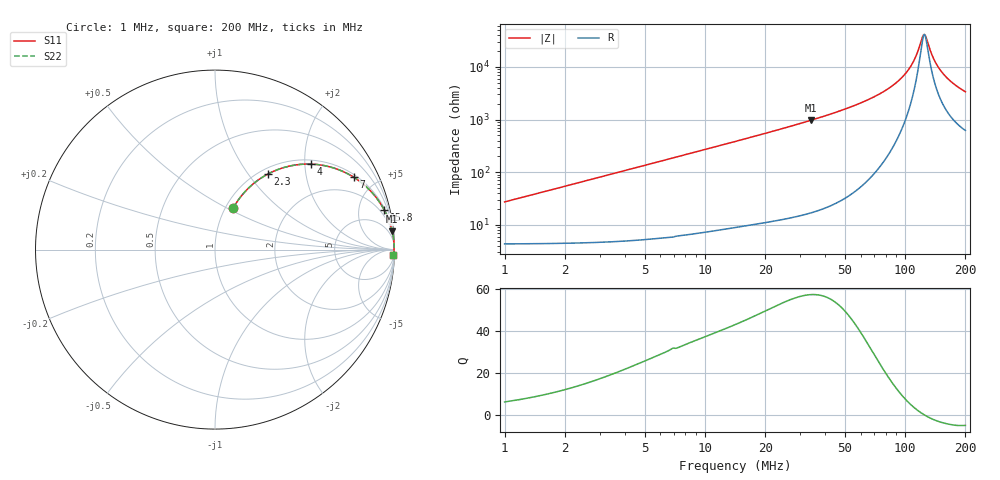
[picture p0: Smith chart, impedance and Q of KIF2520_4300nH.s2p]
!version-2
!date-12.2020
!Series
# MHz S RI R 50
!Freq ReS11 ImS11 ReS21 ImS21 ReS12 ImS12 ReS22 ImS22
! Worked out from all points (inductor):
!   1991 points, 1 MHz to 200 MHz, reference 50 ohm
!   read as one part in series: L = 4.29 uH near 1.9 MHz
!   highest Q = 57.4 at 33.8 MHz (marker M1), where L = 4.56 uH
!   self-resonance near 124.9 MHz
!   S11 on the Smith chart (normalised r, x): 1 MHz: 1.09, +0.54; 2.3 MHz: 1.09, +1.24; 4 MHz: 1.10, +2.16; 7 MHz: 1.12, +3.78; 15.8 MHz: 1.19, +8.57; 200 MHz: 13, -66
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1  0.1019 0.2324  0.8981 -0.2324  0.8981 -0.2324  0.1019 0.2324
2.3  0.2929 0.4201  0.7071 -0.4201  0.7071 -0.4201  0.2929 0.4201
4  0.5371 0.4763  0.4629 -0.4763  0.4629 -0.4763  0.5371 0.4763
5.4  0.6741 0.4506  0.3259 -0.4506  0.3259 -0.4506  0.6741 0.4506
7  0.7743 0.4027  0.2257 -0.4027  0.2257 -0.4027  0.7743 0.4027
10.5  0.8831 0.3084  0.1169 -0.3084  0.1169 -0.3084  0.8831 0.3084
15.8  0.9441 0.219  0.0559 -0.219  0.0559 -0.219  0.9441 0.219
23.7  0.9745 0.1485  0.0255 -0.1485  0.0255 -0.1485  0.9745 0.1485
33.8  0.9877 0.1018  0.0123 -0.1018  0.0123 -0.1018  0.9877 0.1018
34.2  0.988 0.1004  0.012 -0.1004  0.012 -0.1004  0.988 0.1004
67.4  0.9972 0.0395  0.00282 -0.0395  0.00282 -0.0395  0.9972 0.0395
86.9  0.998 0.0223  0.002 -0.0223  0.002 -0.0223  0.998 0.0223
100.5  0.9981 0.0131  0.00195 -0.0131  0.00195 -0.0131  0.9981 0.0131
111.6  0.9979 0.00675  0.00209 -0.00675  0.00209 -0.00675  0.9979 0.00675
121.8  0.9977 0.00149  0.00233 -0.00149  0.00233 -0.00149  0.9977 0.00149
123.8  0.9976 0.000517  0.00239 -0.000517  0.00239 -0.000517  0.9976 0.000517
126.7  0.9975 -0.000869  0.00247 0.000869  0.00247 0.000869  0.9975 -0.000869
133.7  0.9973 -0.00408  0.00271 0.00408  0.00271 0.00408  0.9973 -0.00408
139.7  0.9971 -0.00671  0.00294 0.00671  0.00294 0.00671  0.9971 -0.00671
147  0.9968 -0.00977  0.00325 0.00977  0.00325 0.00977  0.9968 -0.00977
166.9  0.9958 -0.0175  0.00423 0.0175  0.00423 0.0175  0.9958 -0.0175
200  0.9938 -0.0288  0.00624 0.0288  0.00624 0.0288  0.9938 -0.0288
